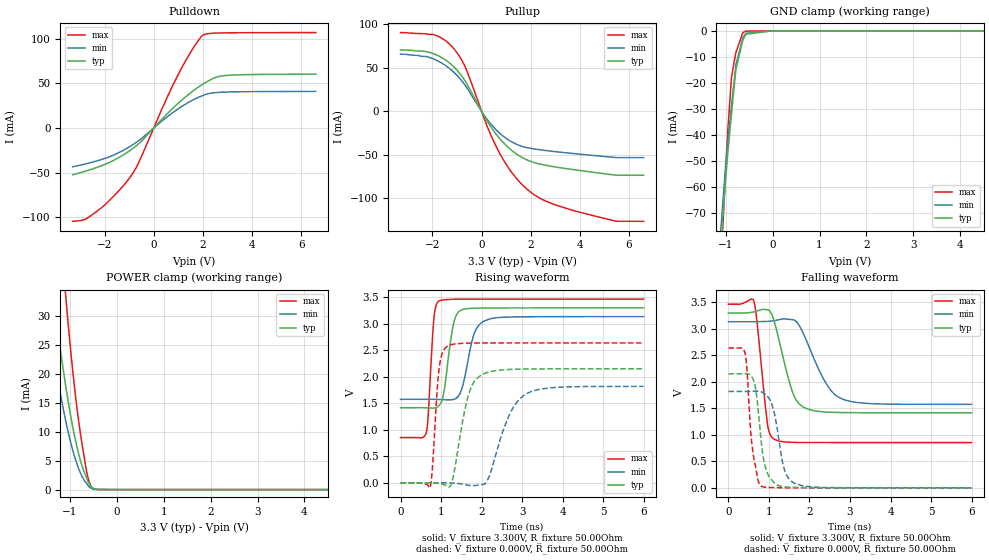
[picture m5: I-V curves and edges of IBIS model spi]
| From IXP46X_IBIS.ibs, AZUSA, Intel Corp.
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[Model]   spi
Model_type   I/O
Vinl = 0.800V
Vinh = 2.000V
Vmeas = 1.500V
Cref = 0.000F
|   typ   min   max
C_comp   3.000pF   2.700pF   3.300pF
[Voltage Range]   3.300V   3.135V   3.465V
[Temperature Range]   25.0   110.0   -40.0
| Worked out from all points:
|   slope of the pulldown table from 0 to 0.495 V, typ, clamps not added: 34.4 ohm
|   slope of the pullup table from 0 to 0.495 V, typ, clamps not added: 22 ohm
|   POWER clamp passes 1 mA (typ) near -0.59 V on its own axis
|   falling waveform, V_fixture 3.300V, R_fixture 50.00Ohm: 20-80 % time 383ps typ, 581ps min, 204ps max; typ from 3.3 V to 1.42 V
|   rising waveform, V_fixture 3.300V, R_fixture 50.00Ohm: 20-80 % time 200ps typ, 269ps min, 115ps max; typ from 1.42 V to 3.3 V
|   rising waveform, V_fixture 0.000V, R_fixture 50.00Ohm: 20-80 % time 330ps typ, 521ps min, 137ps max; typ from 0 V to 2.15 V
|   falling waveform, V_fixture 0.000V, R_fixture 50.00Ohm: 20-80 % time 199ps typ, 255ps min, 166ps max; typ from 2.15 V to 0 V
[Pulldown]
|   Voltage   I(typ)   I(min)   I(max)
-3.3V     -52.46mA   -43.57mA   -104.8mA
-2.775V   -48.45mA   -40.35mA   -102.5mA
-2.275V   -43.93mA   -36.65mA   -92.81mA
-1.545V   -35.07mA   -29.38mA   -74.19mA
-920mV    -24.45mA   -20.02mA   -53.67mA
-605mV    -17.66mA   -14.17mA   -38.56mA
940mV     26.29mA    20.46mA    56.95mA
1.535V    40.21mA    30.6mA     86.58mA
1.99V     49.02mA    36.37mA    104mA
2.545V    57.05mA    39.8mA     106.6mA
2.875V    58.8mA     40.3mA     106.8mA
6.595V    60.44mA    41.09mA    107.2mA
[GND Clamp]
|   Voltage   I(typ)   I(min)   I(max)
-3.3V     -1.837A    -1.782A    -2.189A
-1.11V    -84.94mA   -78.05mA   -94.08mA
-1.01V    -58.95mA   -53.83mA   -56.66mA
-955mV    -47.14mA   -42.92mA   -38.32mA
-875mV    -31.66mA   -28.62mA   -17.74mA
-790mV    -16.23mA   -14.39mA   -8.975mA
-780mV    -14.75mA   -12.96mA   -8.241mA
-635mV    -3.522mA   -2.727mA   -731.8uA
-570mV    -1.397mA   -1.025mA   -117.5uA
0V        -56.84nA   -17.58nA   -565.5pA
6.595V    0A         0A         0A
[Pullup]
|   Voltage   I(typ)   I(min)   I(max)
-3.3V     70.67mA    65.75mA    90.61mA
-1.9V     65.67mA    59.57mA    87.71mA
-1.065V   49.28mA    43.25mA    69.83mA
-630mV    33.14mA    28.45mA    48.54mA
215mV     -10.63mA   -8.762mA   -16.28mA
695mV     -29.83mA   -24.02mA   -46.02mA
1.25V     -45.42mA   -35.42mA   -71.08mA
1.945V    -56.94mA   -42.22mA   -91.7mA
2.785V    -62.85mA   -45.57mA   -105.1mA
3.835V    -67.36mA   -48.7mA    -114.7mA
5.5V      -73.41mA   -53.13mA   -126.3mA
6.595V    -73.41mA   -53.13mA   -126.3mA
[POWER Clamp]
|   Voltage   I(typ)   I(min)   I(max)
-3.3V     221.1mA    178.3mA    361mA
-1.52V    45.83mA    33.1mA     82.51mA
-1.34V    33.02mA    23.22mA    60.37mA
-1.215V   25.09mA    17.21mA    46.38mA
-1.09V    18.05mA    12mA       33.75mA
-930mV    10.52mA    6.586mA    19.92mA
-800mV    5.804mA    3.374mA    11.15mA
-640mV    2mA        1.037mA    3.043mA
-595mV    1.12mA     542.7uA    1.52mA
-540mV    479.4uA    207uA      465.4uA
-390mV    28.44uA    11.22uA    5.344uA
6.595V    0A         0A         0A
[Ramp]
R_load = 50.00Ohm
|   typ   min   max
dV/dt_r   1.291V/329.497ps   1.092V/520.557ps   1.583V/136.841ps
dV/dt_f   1.130V/383.021ps 935.668mV/580.613ps   1.566V/204.115ps
[Falling Waveform]
V_fixture = 3.300V
V_fixture_min = 3.135V
V_fixture_max = 3.465V
R_fixture = 50.00Ohm
|   Time   V(typ)   V(min)   V(max)
0s        3.3V       3.135V     3.465V
630ps     3.321V     3.135V     3.518V
710ps     3.338V     3.135V     3.096V
960ps     3.359V     3.142V     1.22V
1.14ns    3.112V     3.156V     914.3mV
1.58ns    1.811V     3.174V     858.8mV
1.89ns    1.509V     2.841V     855.7mV
2.4ns     1.431V     1.983V     855.9mV
2.79ns    1.421V     1.683V     854.5mV
6ns       1.417V     1.576V     854.3mV
[Rising Waveform]
V_fixture = 3.300V
V_fixture_min = 3.135V
V_fixture_max = 3.465V
R_fixture = 50.00Ohm
|   Time   V(typ)   V(min)   V(max)
0s        1.417V     1.576V     854.3mV
630ps     1.415V     1.576V     938.5mV
820ps     1.41V      1.576V     3.071V
950ps     1.456V     1.573V     3.43V
1.07ns    1.705V     1.568V     3.451V
1.31ns    3.004V     1.574V     3.462V
1.5ns     3.26V      1.743V     3.464V
1.81ns    3.293V     2.798V     3.465V
2.12ns    3.297V     3.068V     3.465V
6ns       3.3V       3.135V     3.465V
[Rising Waveform]
V_fixture = 0.000V
V_fixture_min = 0.000V
V_fixture_max = 0.000V
R_fixture = 50.00Ohm
|   Time   V(typ)   V(min)   V(max)
0s        1.133uV    401.2nV    -5.38nV
730ps     547.1uV    29.42uV    -81.89mV
950ps     -13.29mV   580.4uV    2.146V
1.17ns    -67.05mV   79.97uV    2.582V
1.29ns    82.01mV    -4.105mV   2.613V
1.68ns    1.665V     -45.6mV    2.636V
1.99ns    2.032V     -35.41mV   2.638V
2.71ns    2.14V      1.321V     2.639V
3.05ns    2.146V     1.653V     2.639V
6ns       2.152V     1.819V     2.639V
[Falling Waveform]
V_fixture = 0.000V
V_fixture_min = 0.000V
V_fixture_max = 0.000V
R_fixture = 50.00Ohm
|   Time   V(typ)   V(min)   V(max)
0s        2.152V     1.819V     2.639V
410ps     2.155V     1.819V     2.537V
590ps     2.08V      1.824V     751.1mV
690ps     1.777V     1.826V     310.9mV
810ps     867mV      1.812V     32.28mV
890ps     455.1mV    1.78V      14.03mV
1.03ns    183.9mV    1.651V     7.39mV
1.38ns    19.89mV    344.1mV    1.912mV
1.64ns    8.857mV    84.48mV    392.2uV
6ns       1.133uV    401.2nV    -5.38nV
